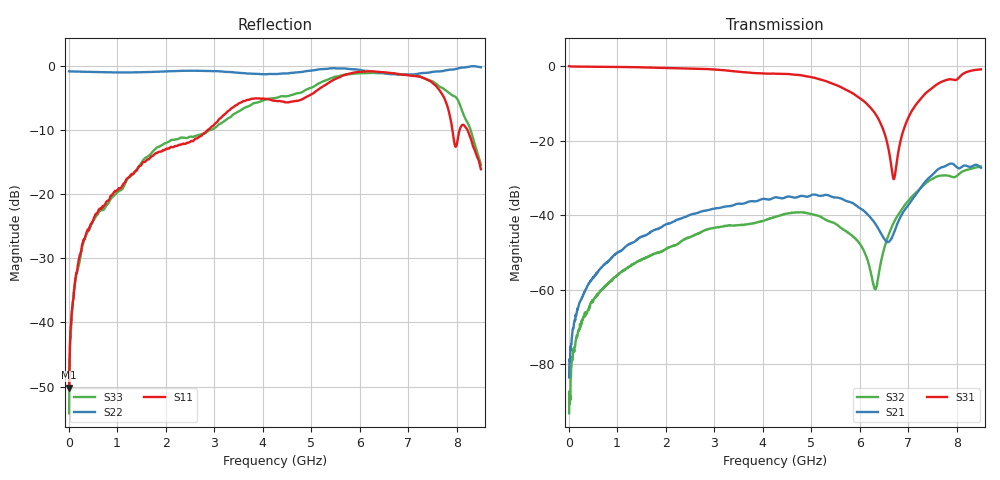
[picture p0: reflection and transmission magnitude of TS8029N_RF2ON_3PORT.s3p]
!Created with skrf (http://scikit-rf.org).
# GHz S RI R 50.0
!freq ReS11 ImS11 ReS12 ImS12 ReS13 ImS13
! ReS21 ImS21 ReS22 ImS22 ReS23 ImS23
! ReS31 ImS31 ReS32 ImS32 ReS33 ImS33
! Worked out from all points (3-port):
!   1601 points, 10 MHz to 8.5 GHz, reference 50 ohm
!   strongest paths, dB at 10 MHz, 2.132 GHz, 4.255 GHz, 6.378 GHz, 8.5 GHz:
!     S31: 0.0, -0.6, -2.1, -13.9, -0.9
!     S21: -83.6, -42.0, -35.3, -43.5, -27.3
!     S32: -93.2, -48.4, -40.5, -57.1, -27.0
!   lowest |S11| = -50.2 dB at 10 MHz (marker M1), VSWR 1.01, Z = 50.1 + j0.304 ohm
!   |S11| at or under -10 dB: start of sweep to 2.872 GHz; 7.913 GHz to 8.062 GHz (148.9 MHz wide, 1.86 % of centre); 8.222 GHz to end of sweep
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0.01  0.000592 0.00304  1.08e-05 4.2e-05  0.9944 -0.00844
      3.15e-05 5.84e-05  -0.9052 0.00355  1e-05 -1.6e-06
      0.9944 -0.00864  5.75e-06 2.11e-05  0.00167 0.00102
0.1426563  0.00879 -0.0205  8.83e-05 0.000418  0.9809 -0.0552
           6.22e-05 0.000454  -0.901 0.0346  6.83e-05 -0.00019
           0.9811 -0.0551  6.62e-05 -0.000189  0.00662 -0.0208
0.6043  -0.00249 -0.073  -0.000128 0.00176  0.9506 -0.219
        -8.23e-05 0.00171  -0.8801 0.1493  -0.0005 -0.000738
        0.9506 -0.219  -0.000504 -0.000727  -0.00865 -0.0699
4.255  -0.5337 0.0249  0.00869 0.0149  -0.0704 -0.7864
       0.00864 0.0149  -0.3225 0.7991  -0.00037 0.00942
       -0.0719 -0.7848  -0.000345 0.00943  -0.5592 -0.0174
5.533806  -0.5826 0.5463  0.0143 0.0096  -0.3671 -0.4082
          0.0143 0.00955  -0.0176 0.9522  0.00552 0.00498
          -0.3679 -0.4082  0.0055 0.00498  -0.5489 0.617
6.319131  -0.2252 0.8727  0.00673 0.00379  -0.2112 -0.094
          0.00673 0.00379  0.0275 0.8899  -0.000235 0.00098
          -0.2114 -0.0933  -0.00023 0.000996  -0.3638 0.7986
6.706487  0.0485 0.871  -0.00152 0.00553  -0.00202 -0.0303
          -0.00151 0.00559  0.161 0.8444  -0.00757 0.00252
          -0.00208 -0.0303  -0.0076 0.00252  0.115 0.8623
7.253031  0.5043 0.6448  -0.00861 0.0212  0.243 -0.2661
          -0.0086 0.0212  0.4024 0.7748  -0.0132 0.0187
          0.2421 -0.2655  -0.0132 0.0187  0.588 0.5751
7.857944  0.4097 0.0341  0.0155 0.0461  0.0938 -0.6565
          0.0156 0.0462  0.5429 0.7564  0.0064 0.0327
          0.0935 -0.658  0.00631 0.0327  0.516 0.3229
8.5  0.1057 0.115  0.023 0.0364  -0.2364 -0.8694
     0.023 0.0364  0.5144 0.8254  0.0177 0.0413
     -0.2376 -0.8688  0.0176 0.0412  0.1684 -0.00709
